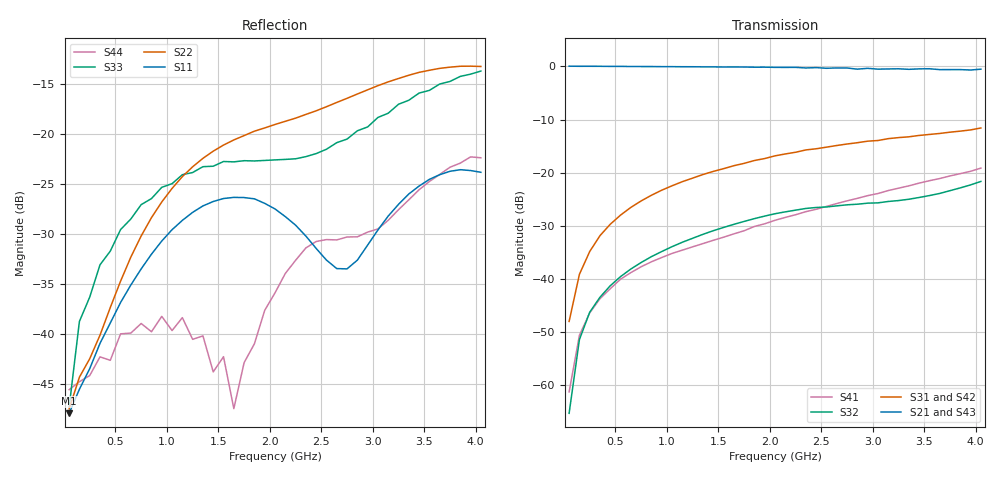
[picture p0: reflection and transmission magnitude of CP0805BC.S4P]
! Network Analyzer HP8720D.07.14 Serial No. US38111185
! 28 Apr 1999  02:06:29
! Frequency 	S11		S21		S31		S41		S12		S22		S23		S24		S13		S23		S33		S34		S14		S24		S34		S44
# HZ  S  DB R 50
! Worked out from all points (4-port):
!   41 points, 50 MHz to 4.05 GHz, reference 50 ohm
!   strongest paths, dB at 50 MHz, 1.05 GHz, 2.05 GHz, 3.05 GHz, 4.05 GHz:
!     S21: 0.0, -0.1, -0.2, -0.5, -0.5
!     S43: 0.0, -0.1, -0.3, -0.8, -0.9
!     S31: -48.0, -22.5, -16.8, -13.9, -11.6
!     S42: -48.8, -22.7, -16.9, -13.9, -11.8
!     S32: -65.3, -33.9, -27.7, -25.7, -21.7
!     S41: -61.3, -35.2, -29.0, -23.9, -19.1
!   lowest |S11| = -48.0 dB at 50 MHz (marker M1), VSWR 1.01, Z = 50.4 - j0.0695 ohm
!   |S11| at or under -10 dB: start of sweep to end of sweep
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5e7  -47.96 -9.9  0.01 -0.8  -48.47 68.0  -62.68 119.9
     0.04 -0.7  -47.53 18.4  -64.61 49.0  -47.61 78.9
     -48.00 95.9  -65.29 117.5  -47.37 28.4  0.01 -1.0
     -61.27 64.6  -48.85 109.2  0.03 -0.8  -45.59 -4.5
1.5e8  -45.55 -48.2  0.03 -2.0  -39.31 87.2  -50.92 82.2
       0.02 -2.1  -44.34 39.4  -50.43 89.0  -39.59 87.2
       -39.13 86.8  -51.42 85.9  -38.76 56.6  0.02 -2.5
       -50.61 89.6  -39.37 87.0  0.02 -2.6  -44.80 25.6
2.5e8  -43.49 -80.3  0.02 -3.4  -34.79 86.2  -46.59 85.6
       0.02 -3.6  -42.50 59.8  -46.31 87.7  -35.07 86.0
       -34.84 85.8  -46.27 87.5  -36.32 56.6  0.01 -4.1
       -46.39 83.8  -35.08 86.1  0.00 -4.3  -44.18 9.3
8.5e8  -32.02 -178.5  -0.03 -11.6  -24.25 76.7  -36.77 77.7
       -0.03 -11.7  -28.36 89.0  -35.83 81.5  -24.54 77.2
       -24.25 76.6  -35.80 81.3  -26.46 46.9  -0.07 -14.0
       -36.77 77.5  -24.52 77.1  -0.05 -14.2  -39.79 13.6
1.65e9  -26.33 123.2  -0.11 -22.3  -18.65 64.9  -31.45 77.9
        -0.11 -22.3  -20.58 51.4  -29.66 73.1  -18.97 66.0
        -18.69 65.6  -29.73 73.3  -22.77 22.2  -0.21 -27.0
        -31.52 78.6  -18.84 66.3  -0.17 -27.0  -47.49 -72.5
2.35e9  -30.21 79.8  -0.24 -31.8  -15.74 54.3  -27.35 74.7
        -0.30 -31.7  -18.02 4.4  -26.67 61.2  -16.07 56.3
        -15.72 55.5  -26.74 61.8  -22.25 0.6  -0.44 -37.9
        -27.34 75.6  -15.81 55.3  -0.47 -38.4  -31.39 -178.1
4.05e9  -23.82 -86.0  -0.56 -56.1  -11.21 31.0  -19.14 47.7
        -0.53 -53.2  -13.22 -81.0  -21.46 57.1  -11.72 35.9
        -11.59 34.8  -21.65 61.5  -13.68 -53.7  -0.84 -65.6
        -19.14 53.3  -11.76 33.6  -0.89 -61.7  -22.36 -2.5
